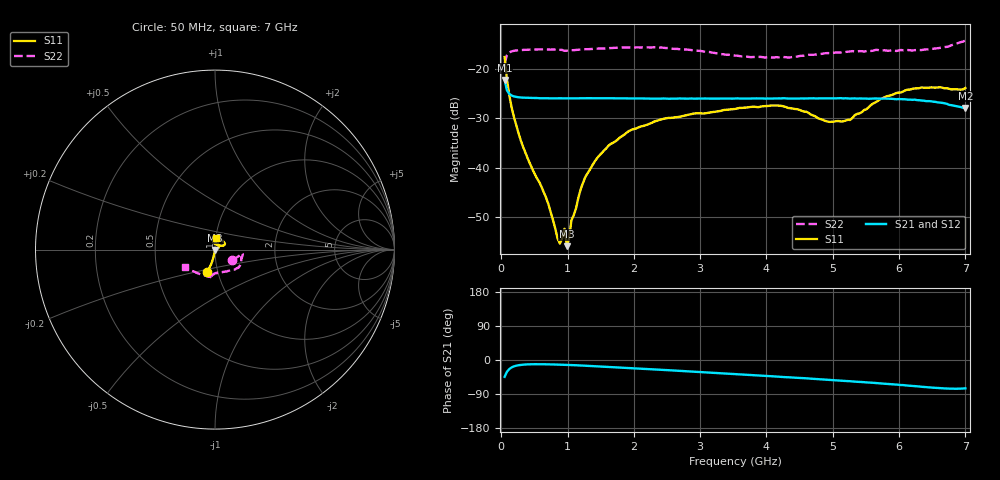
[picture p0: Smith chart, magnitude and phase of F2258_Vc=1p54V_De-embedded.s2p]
! Integrated Device Technology
! Corporate Headquarters
! 6024 Silver Creek Valley Road
! San Jose, CA 95138  USA
! Phone:  1-408-284-8200
! Toll Free:  1-800-223-1366
! Webpage:  http://www.idt.com/
! Timing and RF Division
! 515 Groton Road, Suite 102
! Westford, MA 01886-6024
! Device:  F2258
! Description: Voltage Variable RF Attenuator
! Frequency:  50.0 -  6000.00 MHz
! Package:  3x3 mm Thin QFN Plastic Package: 16 pin
! Ports:  2 RF, 2 DC
!  Pin  1  = NC
!  Pin  2  = NC
!  Pin  3  = RF2  = Port 2
!  Pin  4  = GND
!  Pin  5  = Vdd
!  Pin  6  = NC
!  Pin  7  = VCTRL
!  Pin  8  = NC
!  Pin  9  = GND
!  Pin 10  = RF1  = Port 1
!  Pin 11  = NC
!  Pin 12  = NC
!  Pin 13  = NC
!  Pin 14  = NC
!  Pin 15  = NC
!  Pin 16  = NC
! Vcntrl:  1.540 Volts
! Vdd:  +3.300 Volts
! Current:  1.158 mA
! Data:  The device was measured on a the F2258 evaluation board which has
!  individual transmission lines to the RF pins.  Data was collected
!  using a calibrated network analyzer.  The evaluation board was
!  de-embedded using a TRL calibration technique.
!  The reference plane is the edge of the package pin.
! Misc:  SN 10
!  Action Tracker AT0285
! Date Measured:  2014-12-10
! Date:  2016-01-13  MJV
! Note:
!  Integrated Device Technology supplies this data as a sample of measured
!  data at the package pin for this product.  Your particular data for this
!  product may vary.
!  Data was taken at 25 degrees C.
!  Integrated Device Technology reserves the right to change this data at anytime.
!Freq_(GHz)  S11M_(dB)  S11P_(deg)  S21M_(dB)  S21P_(deg)  S12M_(dB)  S12P_(deg)  S22M_(dB)  S22P_(deg)
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# GHz S dB R 50
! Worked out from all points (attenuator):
!   201 points, 50 MHz to 7 GHz, reference 50 ohm
!   highest |S21| = -22.24 dB at 50 MHz (marker M1); lowest = -27.9 dB at 7 GHz (marker M2)
!   lowest |S11| = -55.8 dB at 988.2 MHz (marker M3), VSWR 1.00, Z = 50 - j0.158 ohm
!   |S11| at or under -10 dB: start of sweep to end of sweep
!   |S22| runs from -18.9 to -14.3 dB; largest |S21 - S12| = 0.00061
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0.05  -17.60 -108.8  -22.24 -44.3  -22.28 -44.4  -18.88 -31.7
0.08475  -22.05 -104.2  -24.31 -31.3  -24.35 -31.3  -17.23 -15.2
0.15425  -27.71 -102.1  -25.37 -19.7  -25.42 -19.8  -16.46 -9.4
0.29325  -34.42 -100.7  -25.78 -13.0  -25.80 -13.0  -16.20 -8.2
0.6755  -46.03 -84.8  -25.92 -11.3  -25.97 -11.3  -16.05 -12.3
0.84925  -54.25 -41.8  -25.93 -12.1  -26.00 -12.1  -16.12 -15.2
0.884  -55.28 -17.0  -25.94 -12.3  -25.98 -12.3  -16.14 -16.1
0.9535  -52.29 -87.3  -25.93 -12.7  -25.96 -12.7  -16.35 -16.6
0.98825  -55.81 -76.8  -25.94 -12.9  -25.95 -12.9  -16.32 -17.5
1.023  -54.26 -31.3  -25.95 -13.2  -25.96 -13.2  -16.26 -18.1
1.05775  -50.58 -13.1  -25.95 -13.4  -25.96 -13.4  -16.22 -18.5
1.2315  -43.05 13.2  -25.93 -14.7  -25.93 -14.7  -16.05 -21.3
1.44  -38.11 16.8  -25.93 -16.8  -25.95 -16.8  -15.92 -24.4
1.6485  -35.17 20.8  -25.94 -18.7  -25.95 -18.7  -15.79 -27.5
2.37825  -30.32 40.5  -26.03 -25.5  -26.03 -25.5  -15.68 -37.9
3.525  -28.09 88.0  -25.98 -37.1  -26.04 -37.1  -17.31 -63.1
4.1505  -27.38 103.6  -25.97 -43.7  -26.01 -43.7  -17.63 -83.1
4.7065  -29.41 93.8  -25.93 -49.7  -25.99 -49.6  -17.16 -94.1
5.2625  -30.31 48.9  -25.99 -55.9  -26.04 -55.9  -16.46 -98.6
5.85325  -25.41 26.3  -26.03 -63.6  -26.11 -63.6  -16.32 -101.8
6.33975  -23.73 32.4  -26.39 -70.7  -26.44 -70.7  -16.20 -113.3
7  -23.86 83.6  -27.87 -74.8  -27.89 -74.9  -14.25 -150.0
